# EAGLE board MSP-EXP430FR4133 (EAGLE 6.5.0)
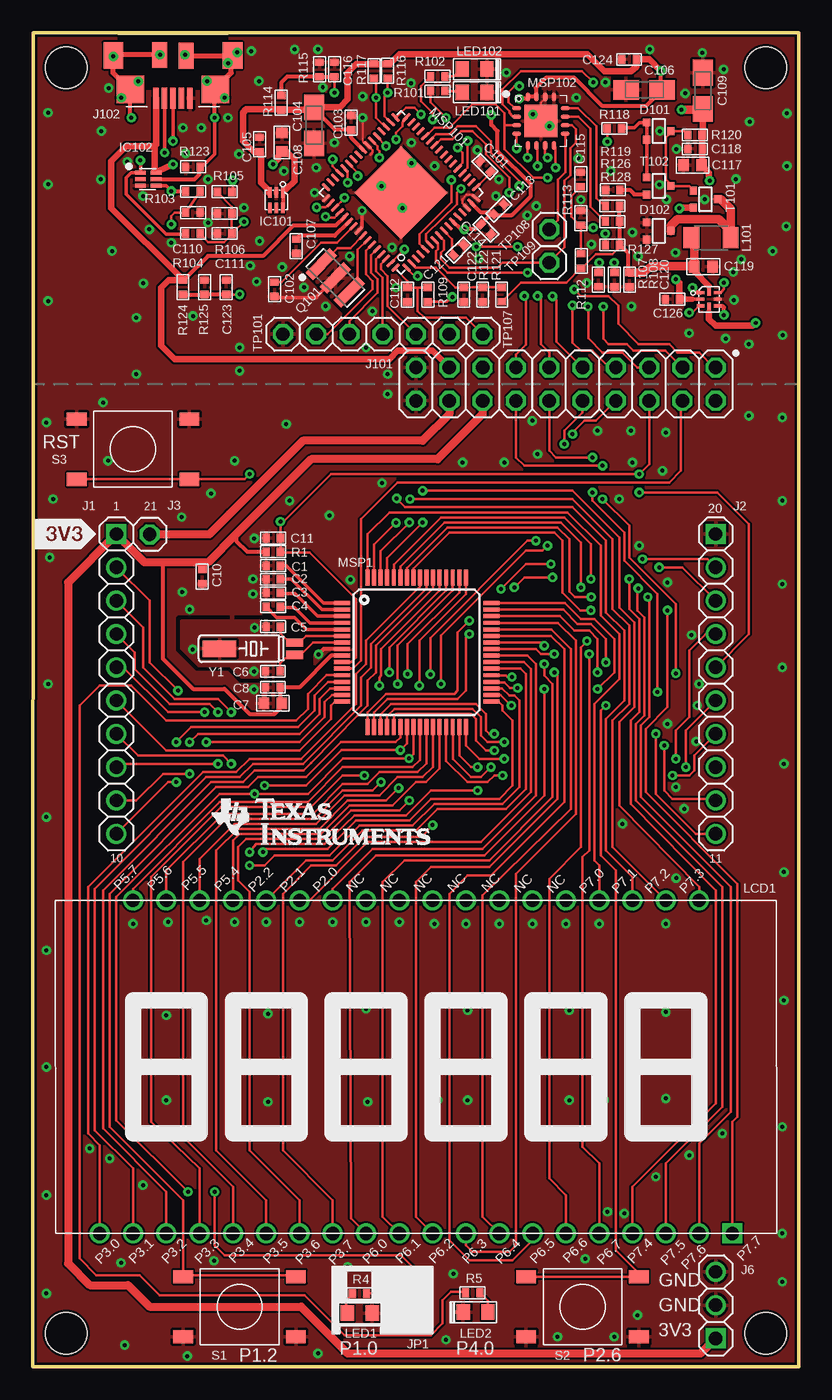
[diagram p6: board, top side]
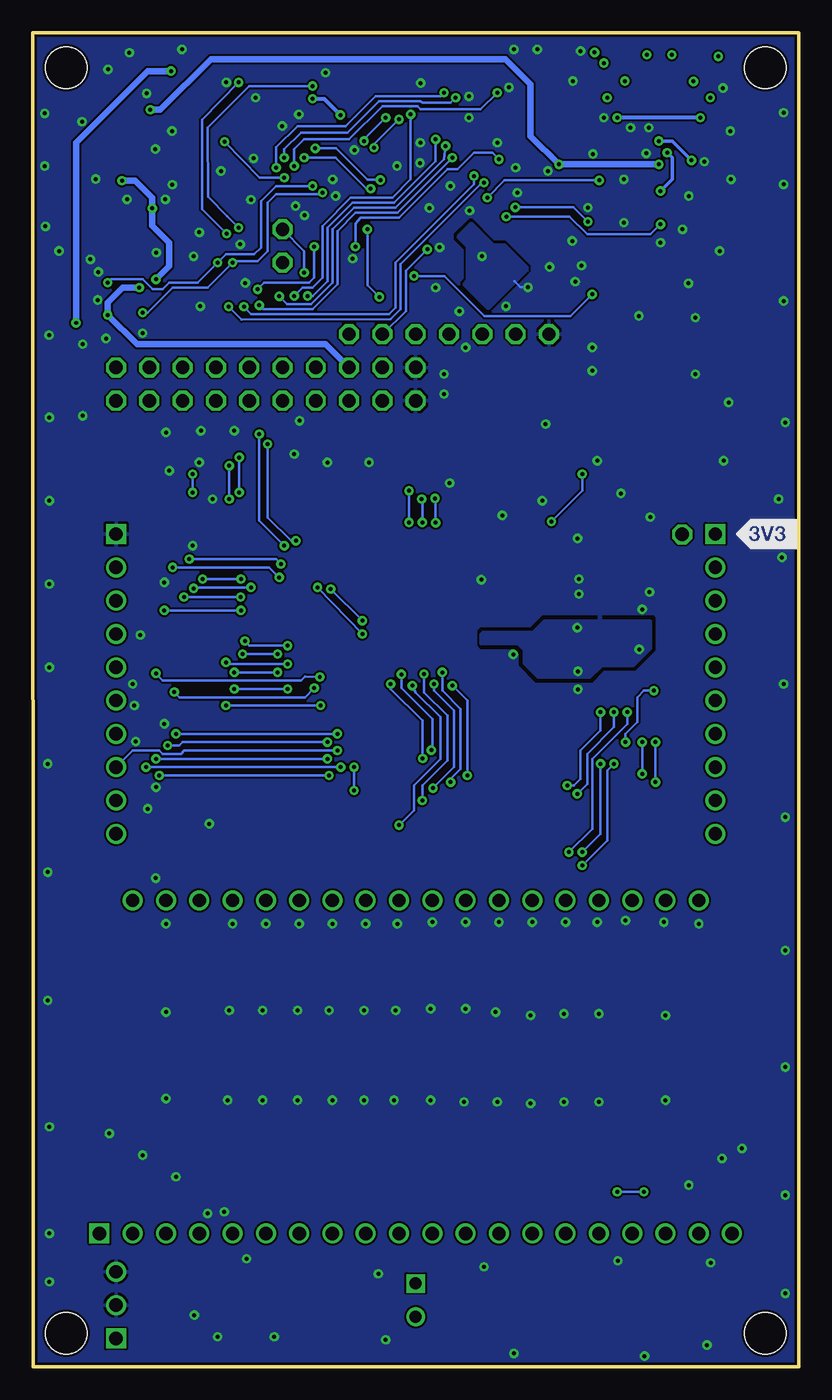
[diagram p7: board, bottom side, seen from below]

Size 58.45 x 101.73 mm. Coordinates in mm from the lower left corner, seen from the top.
Outline: 0,0 58.42,0 58.45,101.73 0.03,101.73 0,0
Copper layers (1*16): Top 0.0178mm / dielectric 12mil / Bottom 0.0178mm
Design rules "default": minimum track width 6mil, minimum drill 12mil, track to track 6mil, track to pad 6mil, pad to pad 6mil, via to via 8mil, smd to smd 0mil, copper to edge 8mil, drill to drill 8mil, minimum pad ring 10mil, minimum via ring 8mil, stop-mask expansion 3mil, vias tented up to drill 15mil, thermal gap 8mil
tRestrict: area 20.5,80.4 to 26.3,87.5; area 10.9,52.2 to 24.5,57.3
bRestrict: area 20.5,80.4 to 26.3,87.5; area 10.9,52.2 to 24.5,57.3

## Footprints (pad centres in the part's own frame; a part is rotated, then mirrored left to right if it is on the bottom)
C0402 = smd 0.55 x 0.65: 1 -0.55,0; 2 0.55,0
C0603 = smd 0.8 x 0.9: 1 -0.7,-0.05; 2 0.7,-0.05
A/3216-18R = smd 1.95 x 1.5: + 1.375,0; - -1.375,0
SOT323 = smd 0.6 x 0.55: 1 -0.65,-0.825; 2 0.65,-0.825; 3 0,1.025
WSON_DSE = smd 0.25 x 0.8: 1 0,0; 2 0.5,0; 3 1,0; 5 0.5,1.15; 6 0,1.15; P4 1,1.15
SON(DRY)6 = smd 0.81 x 0.305: 1 -0.1,0; 2 -0.1,-0.5; 3 -0.1,-1; 4 1.1,-1; 5 1.1,-0.5; 6 1.1,0
UQFN_RSE = smd 0.25 x 0.58: 1 -0.5,-0.65; 2 0,-0.65; 3 0.5,-0.65; 5 0.5,0.65; 6 0,0.65; 7 -0.5,0.65 | smd 0.58 x 0.25: 4 0.55,0; 8 -0.55,0
PINHEAFER1X10 = drill 1.016 square: 1 -11.43,0 | drill 1.016: 2 -8.89,0; 3 -6.35,0; 4 -3.81,0; 5 -1.27,0; 6 1.27,0; 7 3.81,0; 8 6.35,0; 9 8.89,0; 10 11.43,0
1X01 = drill 1.016 octagon: 1 0,0
PINHEADER1X3 = drill 1.016 square: 1 -2.54,0 | drill 1.016: 2 0,0; 3 2.54,0
2X10 = drill 1.016 octagon: 1 -11.43,-1.27; 2 -11.43,1.27; 3 -8.89,-1.27; 4 -8.89,1.27; 5 -6.35,-1.27; 6 -6.35,1.27; 7 -3.81,-1.27; 8 -3.81,1.27; 9 -1.27,-1.27; 10 -1.27,1.27; 11 1.27,-1.27; 12 1.27,1.27; 13 3.81,-1.27; 14 3.81,1.27; 15 6.35,-1.27; 16 6.35,1.27; 17 8.89,-1.27; 18 8.89,1.27; 19 11.43,-1.27; 20 11.43,1.27
EZFET_UX62M-B-5P = smd 0.42 x 1.6: 1 1.3,1.3; 2 0.65,1.3; 3 0,1.3; 4 -0.65,1.3; 5 -1.3,1.3 | smd 2.1 x 2.1: S1 -3.25,0.65; S2 3.25,0.65 | smd 1.5 x 2: S3 -4.55,-1.95; S4 4.55,-1.95 | smd 1.144 x 1.949: S5 -1.016,-1.93; S6 1.016,-1.981
JUMPER-2.54 = drill 0.914 square: 1 0,-1.27 | drill 0.914: 2 0,1.27
L3216C = smd 1.2 x 1.6: 1 -1.5,0; 2 1.5,0
FH1138P = drill 1.016 square: 1 25.4,0 | drill 1.016: 2 22.86,0; 3 20.32,0; 4 17.78,0; 5 15.24,0; 6 12.7,0; 7 10.16,0; 8 7.62,0; 9 5.08,0; 10 2.54,0; 11 0,0; 12 -2.54,0; 13 -5.08,0; 14 -7.62,0; 15 -10.16,0; 16 -12.7,0; 17 -15.24,0; 18 -17.78,0; 19 -20.32,0; 20 -22.86,0; 21 -20.32,25.4; 22 -17.78,25.4; 23 -15.24,25.4; 24 -12.7,25.4; 25 -10.16,25.4; 26 -7.62,25.4; 27 -5.08,25.4; 28 -2.54,25.4; 29 0,25.4; 30 2.54,25.4; 31 5.08,25.4; 32 7.62,25.4; 33 10.16,25.4; 34 12.7,25.4; 35 15.24,25.4; 36 17.78,25.4; 37 20.32,25.4; 38 22.86,25.4
LED0805 = smd 1 x 1.2: A 1.052,0.102; C -0.848,0.102
LQFP64 = smd 1.2 x 0.3: 1 -5.649,3.623; 2 -5.649,3.123; 3 -5.649,2.623; 4 -5.649,2.123; 5 -5.649,1.623; 6 -5.649,1.123; 7 -5.649,0.623; 8 -5.649,0.123; 9 -5.649,-0.377; 10 -5.649,-0.877; 11 -5.649,-1.377; 12 -5.649,-1.877; 13 -5.649,-2.377; 14 -5.649,-2.877; 15 -5.649,-3.377; 16 -5.649,-3.877; 33 5.751,-3.877; 34 5.751,-3.377; 35 5.751,-2.877; 36 5.751,-2.377; 37 5.751,-1.877; 38 5.751,-1.377; 39 5.751,-0.877; 40 5.751,-0.377; 41 5.751,0.123; 42 5.751,0.623; 43 5.751,1.123; 44 5.751,1.623; 45 5.751,2.123; 46 5.751,2.623; 47 5.751,3.123; 48 5.751,3.623 | smd 0.3 x 1.2: 17 -3.699,-5.827; 18 -3.199,-5.827; 19 -2.699,-5.827; 20 -2.199,-5.827; 21 -1.699,-5.827; 22 -1.199,-5.827; 23 -0.699,-5.827; 24 -0.199,-5.827; 25 0.301,-5.827; 26 0.801,-5.827; 27 1.301,-5.827; 28 1.801,-5.827; 29 2.301,-5.827; 30 2.801,-5.827; 31 3.301,-5.827; 32 3.801,-5.827; 49 3.801,5.573; 50 3.301,5.573; 51 2.801,5.573; 52 2.301,5.573; 53 1.801,5.573; 54 1.301,5.573; 55 0.801,5.573; 56 0.301,5.573; 57 -0.199,5.573; 58 -0.699,5.573; 59 -1.199,5.573; 60 -1.699,5.573; 61 -2.199,5.573; 62 -2.699,5.573; 63 -3.199,5.573; 64 -3.699,5.573
RGC64 = smd 0.825 x 0.28: 1 -4.36,3.75; 2 -4.36,3.25; 3 -4.36,2.75; 4 -4.36,2.25; 5 -4.36,1.75; 6 -4.36,1.25; 7 -4.36,0.75; 8 -4.36,0.25; 9 -4.36,-0.25; 10 -4.36,-0.75; 11 -4.36,-1.25; 12 -4.36,-1.75; 13 -4.36,-2.25; 14 -4.36,-2.75; 15 -4.36,-3.25; 16 -4.36,-3.75; 33 4.36,-3.75; 34 4.36,-3.25; 35 4.36,-2.75; 36 4.36,-2.25; 37 4.36,-1.75; 38 4.36,-1.25; 39 4.36,-0.75; 40 4.36,-0.25; 41 4.36,0.25; 42 4.36,0.75; 43 4.36,1.25; 44 4.36,1.75; 45 4.36,2.25; 46 4.36,2.75; 47 4.36,3.25; 48 4.36,3.75 | smd 0.28 x 0.825: 17 -3.75,-4.36; 18 -3.25,-4.36; 19 -2.75,-4.36; 20 -2.25,-4.36; 21 -1.75,-4.36; 22 -1.25,-4.36; 23 -0.75,-4.36; 24 -0.25,-4.36; 25 0.25,-4.36; 26 0.75,-4.36; 27 1.25,-4.36; 28 1.75,-4.36; 29 2.25,-4.36; 30 2.75,-4.36; 31 3.25,-4.36; 32 3.75,-4.36; 49 3.75,4.36; 50 3.25,4.36; 51 2.75,4.36; 52 2.25,4.36; 53 1.75,4.36; 54 1.25,4.36; 55 0.75,4.36; 56 0.25,4.36; 57 -0.25,4.36; 58 -0.75,4.36; 59 -1.25,4.36; 60 -1.75,4.36; 61 -2.25,4.36; 62 -2.75,4.36; 63 -3.25,4.36; 64 -3.75,4.36 | smd 5 x 5: TP 0,0
RSA16 = smd 0.7 x 0.35: 1 -1.85,0.975; 2 -1.85,0.325; 3 -1.85,-0.325; 4 -1.85,-0.975; 9 1.85,-0.975; 10 1.85,-0.325; 11 1.85,0.325; 12 1.85,0.975 | smd 0.35 x 0.7: 5 -0.975,-1.85; 6 -0.325,-1.85; 7 0.325,-1.85; 8 0.975,-1.85; 13 0.975,1.85; 14 0.325,1.85; 15 -0.325,1.85; 16 -0.975,1.85 | smd 2.5 x 2.5: TP 0,0
CSTCR4M = smd 0.8 x 2.6: 1 -1.5,0; 2 0,0; 3 1.5,0
R0402 = smd 0.55 x 0.65: 1 -0.55,0; 2 0.55,0
T062S = smd 1.5 x 1: 1 -4.3,2.3; 2 4.3,2.3; 3 -4.3,-2.3; 4 4.3,-2.3
MOUNTHOLE_125MIL = hole 3.175: 0,0
MS3V-T1R = smd 0.635 x 1.27: P1 -0.47,-4.43; P2 0.47,-4.43 | smd 1.27 x 2.54: P3 0,1.3

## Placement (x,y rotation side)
C1  100n  [C0402]  18.34,61.09 180 top
C2  100n  [C0402]  18.34,60.05 180 top
C3  100n  [C0402]  18.34,59 180 top
C4  1u  [C0402]  18.34,57.96 180 top
C5  12p  [C0402]  18.34,56.44 180 top
C6  12p  [C0402]  18.31,53.04 180 top
C7  10u  [C0603]  18.31,50.55 180 top
C8  100n  [C0402]  18.31,51.82 180 top
C10  100n  [C0402]  12.93,60.25 270 top
C11  1n  [C0402]  18.34,63.2 180 top
C101  470n  [C0402]  34.51,91.53 135 top
C102  220n  [C0402]  18.44,82.17 270 top
C103  100n  [C0402]  24.28,94.87 90 top
C104  10u  [A/3216-18R]  21.46,94.67 90 top
C105  100n  [C0402]  17.3,93.22 90 top
C106  4.7u  [A/3216-18R]  46.63,97.38 0 top
C107  220n  [C0402]  20.09,85.45 270 top
C108  1u  [C0603]  18.95,93.37 90 top
C109  4.7u  [A/3216-18R]  51.11,97.31 270 top
C110  10p  [C0402]  12.22,88.01 0 top
C111  10p  [C0402]  14.63,86.42 180 top
C112  1n  [C0402]  28.58,81.76 270 top
C113  100n  [C0402]  35.55,88.27 45 top
C114  100n  [C0402]  34.57,86.74 315 top
C115  32p  [C0402]  41.81,90.55 270 top
C116  32p  [C0402]  23.01,98.93 270 top
C117  4.7u  [C0603]  50.33,91.57 180 top
C118  100n  [C0402]  50.51,92.88 180 top
C119  4.7u  [C0603]  51.16,83.93 0 top
C120  100n  [C0402]  45.52,82.9 270 top
C121  100n  [C0402]  32.48,85.16 45 top
C122  32p  [C0402]  32.88,81.76 90 top
C123  32p  [C0402]  14.76,82.32 270 top
C124  100n  [C0402]  45.49,99.7 180 top
C126  100n  [C0402]  48.79,81.41 180 top
D101  BAS40-05  [SOT323]  47.65,94.23 270 top
D102  BAS40-05  [SOT323]  47.65,86.61 270 top
DRAW1  [LOGO-ROCKET-10X7MM-BRD]  3.86,81.8 65 top
DRAW3  [LOGO-ROCKET-10X7MM-BRD]  34.15,38.62 7 top
IC101  [WSON_DSE]  19.08,89.53 180 top
IC102  TPD4E004DRYR  [SON(DRY)6]  8.31,91.06 0 top
IC103  TS5A21366RSER  [UQFN_RSE]  51.59,81.41 270 top
J1  [PINHEAFER1X10]  6.38,52.07 270 top
J2  [PINHEAFER1X10]  52.1,52.07 270 top
J3  TEST_PIN2  [1X01]  8.92,63.47 0 top
J6  [PINHEADER1X3]  52.1,4.7 90 top
J101  [2X10]  40.67,74.93 180 top
J102  Micro-USB  [EZFET_UX62M-B-5P]  10.69,98.04 180 top
JP1  [JUMPER-2.54]  29.24,5.08 180 top
L101  2u2  [L3216C]  51.73,86.1 180 top
LCD1  [FH1138P]  27.97,10.16 0 top
LED1  Red  [LED0805]  25.04,4.19 180 top
LED2  Green  [LED0805]  33.68,4.06 0 top
LED101  Red  [LED0805]  33.81,97.28 180 top
LED102  Green  [LED0805]  33.81,99.06 180 top
MSP1  MSP430FR4x  [LQFP64]  29.24,54.61 0 top
MSP101  MSP430F5528IRGC  [RGC64]  28.09,89.54 135 top
MSP102  MSP430G2452IRSA16R  [RSA16]  38.76,95 0 top
Q101  PIEZO_CSTCR4M00G15L99  [CSTCR4M]  23.08,83.02 315 top
R1  47k  [R0402]  18.34,62.15 0 top
R4  470  [R0402]  24.92,5.59 180 top
R5  470  [R0402]  33.55,5.64 0 top
R101  470  [R0402]  30.89,97.28 180 top
R102  470  [R0402]  30.89,98.41 180 top
R103  27  [R0402]  12.22,89.63 0 top
R104  27  [R0402]  12.22,86.42 0 top
R105  1k4  [R0402]  14.63,89.6 0 top
R106  1M  [R0402]  14.63,87.95 180 top
R107  47k  [R0402]  43.15,82.91 270 top
R108  47k  [R0402]  44.37,82.91 270 top
R109  47k  [R0402]  30.14,81.76 270 top
R112  220k  [R0402]  41.84,84.33 90 top
R113  220k  [R0402]  41.81,87.6 90 top
R114  220k  [R0402]  18.95,96.39 90 top
R115  220k  [R0402]  21.87,98.93 90 top
R116  4k7  [R0402]  27.06,98.82 270 top
R117  4k7  [R0402]  26.03,98.82 270 top
R118  820  [R0402]  44.37,94.42 180 top
R119  0  [R0402]  44.24,89.75 180 top
R120  470  [R0402]  50.51,93.94 180 top
R121  220k  [R0402]  35.78,81.76 90 top
R122  220k  [R0402]  34.32,81.76 270 top
R123  33k  [R0402]  12.22,91.5 180 top
R124  240k  [R0402]  11.46,82.32 270 top
R125  150k  [R0402]  13.11,82.32 90 top
R126  2k2  [R0402]  44.22,88.52 180 top
R127  3k3  [R0402]  44.22,85.55 180 top
R128  6k8  [R0402]  44.22,87.33 180 top
S1  T062S  [T062S]  15.77,4.57 180 top
S2  T062S  [T062S]  41.94,4.57 180 top
S3  T062S  [T062S]  7.65,69.98 0 top
T101  DMG1013UW  [SOT323]  51.21,89.03 270 top
T102  BC850CW-115  [SOT323]  47.65,90.04 270 top
TP101  TEST_PIN2  [1X01]  19.08,78.74 0 top
TP102  TEST_PIN2  [1X01]  21.62,78.74 0 top
TP103  TEST_PIN2  [1X01]  24.16,78.74 0 top
TP104  TEST_PIN2  [1X01]  26.7,78.74 0 top
TP105  TEST_PIN2  [1X01]  29.24,78.74 0 top
TP106  TEST_PIN2  [1X01]  31.78,78.74 0 top
TP107  TEST_PIN2  [1X01]  34.32,78.74 0 top
TP108  TEST_PIN2  [1X01]  39.4,86.74 0 top
TP109  TEST_PIN2  [1X01]  39.4,84.2 0 top
U$2  MOUNTHOLE_125MIL  [MOUNTHOLE_125MIL]  2.57,2.54 0 top
U$3  MOUNTHOLE_125MIL  [MOUNTHOLE_125MIL]  2.57,99.06 0 top
U$4  [LOGO16_TPLACE]  13.55,39.64 0 top
U$5  MOUNTHOLE_125MIL  [MOUNTHOLE_125MIL]  55.91,2.54 0 top
U$6  MOUNTHOLE_125MIL  [MOUNTHOLE_125MIL]  55.91,99.06 0 top
U$7  SILK_3V3_TAG  [SILK_3V3_TAG]  0.03,62.36 0 top
U$8  SILK_FR4133_REAR_REV02  [SILK_FR4133_REAR_REV02]  0.03,0.13 0 top
Y1  32.768kHz  [MS3V-T1R]  15.54,54.76 90 top

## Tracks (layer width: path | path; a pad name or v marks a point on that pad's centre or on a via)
5V
  Top 0.152: 8.92,63.5 J3.1
  Top 0.61: J101.18 31.78,72.64 29.74,70.61 20.6,70.61 15.01,65.02 13.46,63.48 J3.1
+3V3
  Top 0.203: 19.01,50.36 C7.1
  Top 0.305: MSP1.9 22.76,54.23 20.35,51.82 C8.1 18.86,50.47 C7.1 19.01,50.57 | 15.52,63.5 15.52,62.98 16.35,62.15 R1.1 | 10.06,61.34 9.93,61.21 9.93,53.98 12.22,51.69 14.63,51.69 16.54,49.78 18.44,49.78 19.01,50.36 | C10.1 12.93,61.34
  Top 0.61: J6.1 50.95,1.02 24.03,1.02 20.47,4.57 8.92,4.57 7.26,6.22 4.34,6.22 2.69,7.87 2.69,59.82 J1.1 8.53,61.34 10.06,61.34 12.93,61.34 13.36,61.34 15.52,63.5 21.23,69.22 30.89,69.22 34.32,72.64 J101.16
EZFET_AVBUS  (via drill 0.3)
  Top 0.203: v29.36,83.19 29.11,83.19 28.52,83.77 MSP101.1 | C123.2 15.38,81.77 v15.77,81.79
  Top 0.305: R124.2 12.96,81.77 12.98,81.79 13.12,81.79 | C123.2 R125.1 13.12,81.79 | 13.23,81.79 13.12,81.79
  Bottom 0.203: v29.36,83.19 27.03,83.19 23.98,80.14 17.42,80.14 v15.77,81.79
EZFET_AVCC  (via drill 0.3)
  Top 0.152: 38.51,93.08 38.51,93.09 MSP102.6
  Top 0.203: 23.01,98.28 v23.01,97.16 | v38.51,91.57 38.51,93.08
  Top 0.305: 23.01,98.28 C116.2 | C116.2 23.01,98.43 22.97,98.38 R115.1 19.41,98.38 18.95,97.92 R114.2 | 23.01,98.3 C116.2 | C116.2 | R114.2
  Bottom 0.203: v23.01,97.16 24.28,95.89 28.85,95.89 29.11,96.14 31.78,96.14 34.32,93.6 37.74,93.6 38.51,92.84 v38.51,91.57
EZFET_AVCCOUT  (via drill 0.3)
  Top 0.152: 36.73,96.01 36.86,96.01 MSP102.1
  Top 0.203: R113.1 41.81,85.98 41.81,84.96 41.83,84.96 R112.2 | R113.1 42.03,86.87 v42.75,86.87 | 36.73,96.01 36.27,96.44 36.27,97.21 36.73,97.66 v37.11,97.66 | 41.78,89.97 41.78,89.94 41.83,89.89 41.86,89.92 | 41.86,89.82 41.86,89.92 | 41.86,89.92 41.86,89.95 41.83,89.97 | C115.2 41.79,90 41.07,89.28 41.07,87.71 41.68,87.1 41.77,86.84 R113.1
  Top 0.508: C115.2 41.78,89.97
  Bottom 0.203: v37.11,97.66 41.94,97.66 45.11,94.49 45.09,89.23 43.61,87.76 v42.75,86.87
EZFET_AVCCOUT2ADC
  Top 0.203: R121.2 34.21,82.31 R122.1 33.59,82.31 C122.2 32.55,82.31 32.25,82.31 30.76,83.82 29.21,83.82 MSP101.2
EZFET_DCDCCAL0
  Top 0.203: R126.2 43.7,88.39 43.33,88.77 42.98,89.13 42.98,94.62 41.6,95.97 MSP102.12
EZFET_DCDCCAL1  (via drill 0.3)
  Top 0.203: MSP102.2 36.85,95.38 36.6,95.38 36.35,95.63 36.35,95.76 35.84,96.27 35.84,97.41 37.24,98.81 41.88,98.81 v42.75,97.94 | R127.2 43.67,85.51 43.66,85.88 43.66,86.34 43.69,86.36 43.66,86.36 v43.66,86.41
  Bottom 0.203: v42.75,97.94 45.54,95.1 45.54,88.27 v43.66,86.41
EZFET_DCDCCAL2
  Top 0.203: R128.2 42.55,88.45 42.55,94.41 41.63,95.33 40.63,95.33 MSP102.11
EZFET_DCDCIO0  (via drill 0.3)
  Top 0.203: v36.91,92.91 36.91,93.15 MSP102.4 | v31.93,90.5 31.93,88.8 29.49,86.36 29.49,85.66 MSP101.5
  Bottom 0.203: v36.91,92.91 35.31,92.91 32.92,90.53 32.16,90.53 v31.93,90.5
EZFET_DCDCIO1  (via drill 0.3)
  Top 0.203: 30.12,85.74 MSP101.6 30,85.86 30,86.36 32.35,88.66 32.36,88.67 32.36,89.53 v32.66,89.84 | v37.74,92.2 37.74,93.11 MSP102.5
  Bottom 0.203: v37.74,92.2 35.33,92.2 32.97,89.84 v32.66,89.84
EZFET_DCDCPULSE  (via drill 0.3)
  Top 0.203: R118.2 43.82,93.72 v43.82,93.42 | v39.27,90.68 38.18,90.68 35.97,92.84 35.97,94.74 | 35.97,94.74 35.97,95.61 35.31,96.27 33.55,96.27 31.78,94.49 30.63,94.49 30,93.86 MSP101.28 | 35.97,94.74 36.04,94.67 MSP102.3
  Bottom 0.203: v39.27,90.68 41.15,90.68 v43.82,93.42
EZFET_DCDCRST  (via drill 0.3)
  Top 0.203: MSP101.7 30.66,85.9 30.91,85.65 30.91,85.24 30.76,85.09 30.76,84.33 31.65,83.44 v37.74,83.44 | 40.78,93.98 MSP102.9 40.61,91.08 40.06,90.53 40.06,87.43 TP108.1 | TP108.1 39.42,86.77 39.37,86.82 TP108.1
  Top 0.305: TP108.1
  Bottom 0.203: TP108.1 | TP108.1 37.74,85.09 v37.74,83.44
EZFET_DCDCTEST
  Top 0.203: MSP101.8 31,86.25 31.37,85.88 31.37,85.19 31.14,84.96 31.14,84.46 31.78,83.82 35.46,83.82 35.84,84.2 TP109.1 39.8,84.61 40.56,85.37 40.56,90.45 41,90.88 41,92.91 41.43,93.34 41.43,94.36 41.12,94.67 40.74,94.67 40.67,94.74 40.67,94.62 MSP102.10
EZFET_DM  (via drill 0.3)
  Top 0.203: J102.2 10.04,96.66
  Top 0.254: IC102.4 10.17,90.06 v10.57,89.66 | 10.04,96.66 v10.06,92.58
  Top 0.305: v10.57,89.66 11.58,89.66 11.61,89.63 R103.1
  Bottom 0.254: v10.57,89.66 9.68,90.55 9.68,92.2 v10.06,92.58
EZFET_DP  (via drill 0.3)
  Top 0.254: v8.2,92 v8.21,92.01 IC102.1 7.52,91.06 7.14,90.68 7.14,89.41 10.19,86.36 11.5,86.36 R104.1 | J102.3 v10.69,93.47
  Bottom 0.254: v10.69,93.47 9.68,93.47 v8.2,92
EZFET_HOSTSCL  (via drill 0.3)
  Top 0.152: MSP101.35 26.95,94.62 26.95,94.61
  Top 0.203: 26.95,94.61 26.83,94.61 26.19,95.25 v26.19,96.77 26.19,98.25 | v39.27,92.2 39.09,92.36 MSP102.7
  Top 0.305: 26.19,98.25 R117.2
  Bottom 0.203: v26.19,96.77 26.57,96.39 28.73,96.39 28.85,96.52 32.03,96.52 34.44,94.11 38,94.11 39.27,92.84 v39.27,92.2
EZFET_HOSTSDA  (via drill 0.3)
  Top 0.203: MSP101.34 27.28,94.92 26.82,95.38 26.82,96.9 v27.08,97.16 27.08,98.16 R116.2 | MSP102.8 39.88,92.98 v39.88,91.44
  Bottom 0.203: v27.08,97.16 27.33,96.9 32.28,96.9 34.57,94.62 38.25,94.62 39.88,92.99 v39.88,91.44
EZFET_LED0  (via drill 0.3)
  Top 0.203: MSP101.20 33.17,91.44 v33.17,93.47 | v31.52,95.25 30.34,96.44 R101.2
  Bottom 0.203: v33.17,93.47 33.17,93.6 v31.52,95.25
EZFET_LED1  (via drill 0.3)
  Top 0.203: R102.2 30.24,98.28 29.62,97.66 29.62,96.52 30.51,95.63 v30.51,95.12 | MSP101.21 32.41,91.44 32.79,91.82 32.79,92.58 v32.41,92.96
  Bottom 0.203: v32.41,92.96 32.41,93.22 v30.51,95.12
EZFET_NC_TMSC  (via drill 0.3)
  Top 0.203: J101.1 51.97,76.2 50.83,77.34 49.17,77.34 48.54,77.98 46.2,77.98 44.65,79.53 44.65,80.92 43.92,81.66 41.81,81.66 v41.3,82.17 | MSP101.45 22.89,91.57 v22.89,92.08 | 36.98,85.47 v36.98,85.42 36.98,85.34 36.93,85.42 v33.83,85.42
  Bottom 0.203: v22.89,92.08 23.39,92.58 24.79,92.58 26.06,91.31 26.82,91.31 30.51,87.63 33.43,87.63 33.83,87.17 v33.83,85.42 | v36.98,85.42 36.98,83.06 37.36,82.68 40.79,82.68 v41.3,82.17
EZFET_PU.0/DP  (via drill 0.3)
  Top 0.152: 22.76,88.77 MSP101.50
  Top 0.203: v16.1,87.33 15.33,86.55 C111.1 | R105.1 15.18,88.48 R106.1 15.18,87.47 C111.1 | R104.2 13.39,85.78 14.58,85.78 15.15,86.35 C111.1 | 22.76,88.77 22.5,88.52 22.45,88.52 22.35,88.42 v21.64,88.42
  Bottom 0.203: v16.1,87.33 17.2,88.42 v21.64,88.42
EZFET_PU.1/DM  (via drill 0.3)
  Top 0.203: R103.2 12.74,89.56 C110.1 10.82,88.01 10.57,87.76 v10.57,87.12 | MSP101.52 23.01,87.63 22.5,87.63 v22.33,87.71
  Bottom 0.203: v22.33,87.71 17.5,87.71 16.15,86.36 11.33,86.36 v10.57,87.12
EZFET_PUR  (via drill 0.3)
  Top 0.203: MSP101.51 23.52,88.85 v23.77,89.15 | v15.24,90.48 15.25,89.7 R105.2
  Bottom 0.203: v15.24,90.48 22.45,90.48 v23.77,89.15
EZFET_RST
  Top 0.203: MSP101.64 27.79,83.62 28.6,82.8 28.6,82.37 C112.1 R109.1 | TP107.1 33.05,80.01 29.87,80.01 29.36,80.52 29.36,82.3 30.12,82.3 R109.1 | R109.1 | R109.1 30.12,82.3
EZFET_SBWTCK  (via drill 0.3)
  Top 0.203: MSP101.44 23.75,91.39 24.03,91.11 v24.03,90.3 | J101.3 48.26,77.47 45.82,77.47 45.31,77.98 43.92,77.98 43.51,78.38 v43.51,80.85
  Bottom 0.203: v24.03,90.3 24.28,90.17 30.38,84.07 30.38,80.65 31.14,79.88 42.52,79.86 v43.51,80.85
EZFET_SBWTDIO  (via drill 0.3)
  Top 0.203: MSP101.43 24.79,91.06 v24.79,90.81 | J101.5 46.13,76.2 44.98,77.34 43.46,77.34 42.37,78.44 42.37,80.82 v42.34,80.85
  Bottom 0.203: v24.79,90.81 24.79,90.17 30.76,84.2 30.76,80.77 31.27,80.26 41.78,80.29 v42.34,80.85
EZFET_SHIELD  (via drill 0.3)
  Top 0.152: 14,97.03 13.87,96.9 13.87,96.77
  Top 0.203: 7.44,95.12 7.52,95.12 v7.52,95.25 | 7.44,96.77 7.39,96.77 | 7.39,96.77 7.39,97.28 | v6.76,96.77 7.39,96.77 | v14.63,96.77 13.87,96.77
  Top 0.254: R123.1 12.92,91.5 13.87,92.46 v13.87,95.25
  Top 0.305: IC102.5 12.21,90.56 12.34,90.55 12.73,90.93 12.73,91.34 R123.1 12.73,91.23 | 7.44,95.12 7.44,96.77 | v13.87,95.25 13.87,96.77
  Top 0.381: J102.S2 7.41,97.39 6.12,98.68 6.12,99.95 6.14,99.97 J102.S4 | J102.S4 v6.14,99.93 v6.15,99.92 | 14,97.03 14,97.45 | J102.S2 7.44,97.33 7.39,97.28 | v8.05,98.02 8.05,98 J102.S2 | v13.28,98.04 v13.29,98.04 J102.S1 14,97.45 | 14,97.45 14,97.54 15.14,98.68 15.14,99.16 v14.88,99.42 14.88,99.64 J102.S3 | v15.6,100.23 15.6,99.97 J102.S3 | J102.S3 15.22,99.97 J102.S5 11.68,99.97 v11.61,100.05 | 9.68,100.05 6.2,100.05 J102.S4
  Top 0.406: J102.S6 9.68,100.05 v9.7,100.05
  Bottom 0.305: v7.52,95.25 v13.87,95.25
EZFET_TCK  (via drill 0.3)
  Top 0.203: v28.35,85.22 27.31,84.18 MSP101.63
  Bottom 0.203: v28.35,85.22 29.97,83.59 29.97,80.49 TP106.1 | TP106.1
EZFET_TDI
  Top 0.203: MSP101.61 26.59,84.86 26.19,84.46 26.19,83.57 26.7,83.06 TP104.1 | TP104.1
EZFET_TDO
  Top 0.203: TP103.1 24.16,79.76 26.31,81.92 26.31,82.93 25.81,83.44 25.81,84.77 MSP101.60
EZFET_TEST
  Top 0.203: 25.93,85.6 25.92,85.6 MSP101.59 25.43,85.1 25.43,83.31 25.93,82.8 25.93,82.17 22.5,78.74 TP102.1
EZFET_TMS
  Top 0.203: MSP101.62 26.95,84.46 26.57,84.07 26.57,83.69 27.08,83.19 27.08,80.9 TP105.1
EZFET_UARTCTS  (via drill 0.3)
  Top 0.203: 28.35,95.12 28.22,94.87 28.22,94.62 27.71,94.11 v27.71,93.6 | 37.62,81.53 v37.49,81.66 37.62,81.53 | J101.13 36.86,77.19 37.62,77.95 37.62,81.53
  Top 0.254: MSP101.32 28.49,95.27 28.35,95.12
  Bottom 0.203: v27.71,93.6 27.71,91.95 30.89,88.77 34.06,88.77 35.97,86.87 35.97,82.8 37.11,81.66 v37.49,81.66
EZFET_UARTRTS  (via drill 0.3)
  Top 0.203: 27.69,95.27 27.71,95.25 | 27.84,95.12 27.71,95.25 | 27.71,95.25 28.47,96.01 29.11,96.01 v29.62,95.5 | J101.11 39.4,77.34 38.76,77.98 38.76,81.41 v38.51,81.66
  Top 0.254: MSP101.33 27.69,95.27
  Bottom 0.203: v29.62,95.5 29.62,90.55 31.01,89.15 34.19,89.15 36.35,87 36.35,83.06 37.11,82.3 37.87,82.3 v38.51,81.66
EZFET_UARTRXD  (via drill 0.3)
  Top 0.203: MSP101.38 26.31,93.09 26.31,92.84 26.44,92.71 v26.44,92.2 | J101.7 43.97,76.2 42.7,77.47 41.81,77.47 41.17,78.11 v41.17,80.95
  Bottom 0.203: v26.44,92.2 30.63,88.01 33.81,88.01 35.2,86.61 35.2,82.55 37.11,80.65 40.87,80.65 v41.17,80.95
EZFET_UARTTXD  (via drill 0.3)
  Top 0.203: MSP101.37 26.25,93.79 v26.95,93.09 | J101.9 39.95,78.18 39.95,81.33 v39.65,81.64
  Bottom 0.203: v26.95,93.09 27.08,92.08 30.76,88.39 33.93,88.39 35.59,86.74 35.59,82.68 37.24,81.03 39.04,81.03 v39.65,81.64
EZFET_V18
  Top 0.203: MSP101.55 24.45,86.96 23.22,85.73 22,85.73 18.99,82.72 C102.1
EZFET_VBUS  (via drill 0.3)
  Top 0.203: 9.3,91.19 9.3,91.06 IC102.6 | 9.55,91.19 IC102.6 | IC102.6 | 51.1,95.66 51.1,95.93 C109.+
  Top 0.254: IC103.2 50.32,81.41
  Top 0.305: MSP101.53 23.11,87.02 19.86,87.02 17.55,84.71 13.36,84.71 11.71,83.06 11.33,83.06 | 19.33,89.79 IC101.1 IC101.6
  Top 0.406: 50.32,81.41 C126.1 49.3,81.41
  Top 0.508: 9.3,93.09 9.3,91.19 | 9.55,91.19 v10.69,91.69 | J101.17 30.51,77.47 27.84,77.47 27.2,76.84 10.82,76.84 9.8,77.85 9.8,82.3 10.38,82.87 R124.1 11.33,83.06 5.99,88.37 5.99,91.95 7.14,93.09 9.3,93.09 | v18.31,91.69 18.69,92.08 18.69,92.33 19.08,92.71 19.04,92.71 C108.1 19.37,92.67 19.96,92.08 19.96,90.42 19.33,89.79 | J102.1 9.39,93.19 9.3,93.09 | 51.1,95.66 51.1,94.01 51.06,93.96 R120.1 C118.1 51.06,91.65 C117.1 51.59,91.06 51.59,90.42 51.61,90.42 v51.64,90.45 | T101.2 49.32,88.38 | 49.32,88.38 49.3,88.39 | v49.33,88.34 49.33,88.37 49.32,88.38 | v49.05,82.93 49.3,82.68 49.3,81.45 C126.1
  Top 0.635: C109.+ 50.62,95.88 50.39,95.86 v49.48,95.86
  Bottom 0.305: 48.87,95.81 48.74,95.86
  Bottom 0.508: v10.69,91.69 v18.31,91.69 20.47,93.85 20.47,97.79 22.38,99.7 44.86,99.7 48.74,95.86 v49.48,95.86 | v51.64,90.45 50.62,90.45 49.33,89.15 v49.33,88.34 49.33,87.02 48.03,85.73 48.03,83.95 v49.05,82.93
EZFET_VCC  (via drill 0.3)
  Top 0.152: MSP101.11 32.03,87.38 32.07,87.34 | 33.86,86.79 C114.1 | 33.43,88.77 MSP101.15
  Top 0.203: 24.66,93.32 MSP101.40 | v32,81.59 31.58,81.21 R109.2 | R116.1 27.08,99.44 | C114.1 34.06,87.12 | 33.86,86.79 34.13,87.06 | 34.95,94.74 34.98,94.77
  Top 0.254: 17.93,89.53 IC101.3 | IC103.4 51.59,80.39
  Top 0.305: MSP101.40 25.19,92.82 24.28,93.73 C103.1 23.05,94.32 21.49,95.89 21.49,96.01 C104.+ | 25.52,99.34 R117.1 25.44,99.31 | 46.17,99.73 C124.1 46.04,99.2 45.99,99.1 | 48.14,97.71 C106.+ | 43.59,98.81 45.69,98.81 45.99,99.1 | 38.42,96.82 38.38,97.03 38.38,97.54 39.14,98.3 41.3,98.3 43.46,96.14 46.76,96.14 47.56,96.93 C106.+ | 38.42,96.82 38.43,96.75 | 33.6,88.61 MSP101.15 | 32.07,87.34 32.66,86.74 v32.92,86.74 33.76,86.74 34.13,87.06 35.08,88.01 | v37.11,96.7 37.64,96.7 MSP102.16 MSP102.15 38.42,96.82 | C106.+ 47.73,97.38 47.9,97.59 v47.9,98.81 | 46.06,99.05 45.99,99.1 | 35.08,88.01 35.38,87.83 36.55,87.83 38,89.28 38,90.17 35.46,92.71 35.46,94.23 34.98,94.72 34.98,94.77 v34.98,95.45 | 35.08,88.01 35.14,88.01 C113.1 | 35.08,88.01 34.19,88.01 33.43,88.77
  Top 0.406: 17.85,89.88 17.93,89.75 17.93,89.53 | 17.42,92.46 17.3,92.46 C105.1 17.3,92.62 16.88,92.62
  Top 0.508: 16.88,92.62 16.03,93.47 16.03,95.63 16.28,95.89 18.91,95.89 R114.1 21.26,95.84 C104.+ 23.42,96.04 24.03,96.65 24.03,98.68 24.66,99.31 25.44,99.31 27,99.31 R116.1 27.26,99.37 27.97,100.08 42.32,100.08 43.59,98.81 45.62,98.81 46.02,99.14 46.02,99.64 | 17.85,89.88 17.42,90.3 17.42,92.46 17.34,92.67 17.35,92.67 | v47.9,98.81 47.02,99.7 C124.1 | v55.14,79.6 55.14,79.63 54.89,79.38 52.1,79.38 51.59,79.88 51.59,80.39
  Bottom 0.203: v32.92,86.74 32.92,82.5 v32,81.59
  Bottom 0.305: v37.11,96.7 36.22,96.7 v34.98,95.45
  Bottom 0.508: v47.9,98.81 49.68,98.81 55.14,93.34 v55.14,79.6
EZFET_VCCEN1  (via drill 0.3)
  Top 0.203: MSP101.26 30.69,93.15 31.14,93.6 32.03,93.6 32.66,94.23 33.55,94.23 34.57,93.22 34.57,92.46 36.35,90.68 v36.35,89.53 | v50.06,80.39 50.32,80.39 50.83,80.91 IC103.3 | R107.1 43.15,83.88 v43.21,84.2
  Bottom 0.203: v36.35,89.53 36.47,89.41 39.9,89.41 40.54,88.77 40.54,85.09 41.3,84.33 43.08,84.33 v43.21,84.2 45.11,82.3 47.78,82.3 49.68,80.39 v50.06,80.39
EZFET_VCCEN2  (via drill 0.3)
  Top 0.203: MSP101.27 30.29,93.51 30.76,93.98 31.78,93.98 32.41,94.62 33.81,94.62 34.95,93.47 34.95,92.58 37.11,90.42 v37.11,90.04 | R108.1 v44.35,84.2 | IC103.7 52.47,81.91 52.73,82.17 v52.73,82.68
  Bottom 0.203: v37.11,90.04 39.9,90.04 41.05,88.9 41.05,85.34 41.55,84.84 43.71,84.84 v44.35,84.2 45.87,82.68 48.03,82.68 48.54,82.17 49.3,82.17 50.06,82.93 52.48,82.93 v52.73,82.68
EZFET_VCCOUT
  Top 0.203: R121.1 35.93,81.37 37.24,82.68 40.69,82.68 41.81,83.81 | 41.81,83.81 41.81,83.82 41.94,83.82 42.95,84.84 44.22,84.84 44.73,85.34 44.73,85.38 R127.1 | 41.81,83.81 R112.1
  Top 0.254: 51.59,82.42 IC103.8
  Top 0.305: R126.1 44.74,88.01 R128.1 R127.1 45.4,84.96 45.4,83.45 C120.1 | 46.63,83.48 46.63,83.45
  Top 0.508: 50.55,83.92 50.55,83.46 51.59,82.42
  Top 0.635: 46.63,83.48 47.19,83.92 50.43,83.92 C119.1 50.46,83.9 50.47,83.9 | L101.2 50.44,85.82 50.44,84.18 50.42,84.18 50.42,84.07 50.55,84.07 50.55,83.92 50.47,83.92 50.47,83.9 | 50.47,83.87 50.47,83.9 | 46.63,83.45 C120.1
EZFET_VCCTARGET  (via drill 0.3)
  Top 0.254: IC103.5 52.21,80.91
  Top 0.305: IC103.1 50.71,81.91 v50.32,82.3 | 52.21,80.91 52.6,80.91 52.73,80.77 v52.73,80.21
  Bottom 0.508: J101.15 36.09,77.98 50.5,77.98 v52.73,80.21 52.73,81.15 51.59,82.3 v50.32,82.3
EZFET_VCORE
  Top 0.203: MSP101.17 34.93,91.07 C101.1
EZFET_VREF
  Top 0.203: C121.1 31.98,84.75 31.98,86 MSP101.9
EZFET_VUSB
  Top 0.305: MSP101.54 23.04,86.25 20.36,86.25 20.09,85.98 | C107.1 20.09,85.98 | 20.09,85.98
EZFET_XT2IN
  Top 0.203: MSP101.57 25.16,86.27 24.23,85.32 23.24,85.32 22.06,84.14 22,84.07
  Top 0.406: Q101.1 22.06,84.08 22.06,84.14
EZFET_XT2OUT
  Top 0.203: MSP101.58 24.79,85.17 24.79,82.8 24.2,82.21
  Top 0.406: Q101.3 24.2,81.96 24.2,82.21
GND  (via drill 0.3)
  Top 0.152: v25.17,95.25 25.17,93.47 25.43,93.22 MSP101.39 | MSP102.TP 38.76,96.39 39.14,96.77 MSP102.14 | 26.79,88.05 26.82,88.01 MSP101.TP 27.2,88.65
  Top 0.203: 33.63,89.31 33.53,89.31 | 33.63,89.31 33.63,89.3 MSP101.16 | MSP101.56 24.83,86.66 | MSP101.39 25.93,92.76 25.93,92.61 25.76,92.43 | MSP101.14 32.79,88.72 32.79,89.05 33.1,89.38 33.53,89.38 33.63,89.31
  Top 0.254: 24.83,86.66 24.86,86.66 25.12,86.92 v25.12,88.16 | Q101.2 22.95,82.9 21.62,81.56
  Top 0.305: 21.62,81.56 18.46,81.53 C102.2 | MSP1.8 22.45,54.73 22.2,54.74 v21.79,54.33
  Bottom 0.203: v20.68,82.32 21.23,82.32 21.72,82.8
  other vias: 10.57,85.73 8.89,86.74 51.08,100.2 41.45,96.77 24.18,84.68 33.91,92.79 35.33,89.28 19.96,100.46 23.01,93.34 53.49,81.36 43.69,97.94 46.18,84.68 45.75,86.51 47.83,94.23 44.09,91.19 52.7,98.93 17.25,98.04 47.07,100.46 35.56,90.55 48.34,89.03 49.1,92.86 8.43,82.63 16.59,83.97 25.17,96.88 28.85,97.89 17.07,82.75 22.35,80.87 19.02,83.87 27.08,74.17 27.41,85.37 30.66,91.57 12.22,80.14 22.12,97.56 5.18,90.55 5.23,94.23 16.66,100.33 5.79,97.51 15.72,92.48 13.36,87.25 11.66,92.53 14.88,95.25 16.1,88.39 8.41,89.28 11.46,94.49 27.71,82.3 47.8,90.14 38.4,88.52 41.61,92.15 42.62,85.6 49.76,97.1 21.62,91.44 41.81,89 7.9,80.01 48.29,71.25 48.41,59.82 45.62,71.37 43.08,71.37 38.1,72.14 1.17,81.28 1.17,90.17 1.17,95.63 21.74,100.46 46.13,3.94 57.18,6.48 57.18,10.16 57.18,53.34 57.18,59.69 57.18,66.04 57.18,72.39 57.2,78.66 57.48,86.97 57.53,91.57 57.53,95.58 54.69,94.95 56.44,85.09 54.64,77.98 54.64,72.52 11.35,64.8 19.33,71.88 46.25,62.61 13.23,34.04 15.39,33.91 17.81,33.91 20.35,33.91 22.89,33.91 25.43,33.91 27.97,33.91 30.63,33.78 33.05,33.78 35.59,33.78 38.13,33.78 40.67,33.78 43.21,33.78 43.84,11.81 45.11,11.68 48.29,33.78 44.98,41.4 22.63,64.92 7.65,33.78 10.31,33.91 10.19,20.32 10.19,26.8 15.27,26.92 15.27,20.19 17.93,20.19 17.93,26.92 20.47,26.8 20.47,20.07 23.14,27.05 23.01,20.19 25.43,27.31 25.55,20.19 28.09,27.31 28.09,20.32 30.76,27.18 30.89,20.32 33.17,27.18 33.17,20.32 35.84,27.18 35.59,20.32 38.25,27.18 38.25,20.32 40.92,27.18 40.92,20.32 43.46,27.18 43.59,20.32 48.29,27.05 48.29,20.45 8.41,13.84 5.87,15.88 4.34,16.64 52.6,17.78 50.06,16.13 47.52,14.48 48.41,49.02 50.6,47.68 49.05,44.2 49.68,42.55 15.39,69.09 19.58,66.04 7.01,1.65 11.79,0.81 21.74,1.02 1.04,5.59 1.04,13.08 1.04,22.86 1.04,31.75 1.04,41.91 1.17,52.07 1.3,61.72 1.04,72.01 40.03,2.29 44.35,2.29 32.08,7.09 24.03,7.62 13.82,8.08 6.73,7.92 42.14,8.23 57.18,18.29 57.3,27.94 57.3,37.72 57.3,45.97 16.79,58.93 16.79,60.07 49.07,37.26 50.83,52.07 50.24,55.8 44.73,66.17 38.51,69.6 35.97,68.96 5.36,73.53 32.79,68.96 1.55,66.17 11.4,59.08 25.43,77.72 27.08,75.69 15.77,77.72 15.77,75.95 7.9,75.69 45.75,68.96 25.91,80.49 48.03,68.33 5.74,69.09 13.59,66.6 50.7,50.42 31.52,2.06 16.89,63.17 11.96,57.76 16.87,51.66 16.87,53.04 12.19,54.71 16.92,56.36 6.05,85.09 19.15,91.19 17.3,85.85 26.59,90.04 28.19,88.37 38.15,95.5 39.42,94.62 21.49,89.53 7.21,91.9 12.85,94.49 13.36,90.55 28.91,91.8 53.64,90.58 37.72,87.81 34.04,84.51 52.86,78.41 49.02,84.96 54.05,84.46 50.06,78.82 53.44,83.49 45.67,80.87 26.64,67.39 24.23,60.02 51.26,89.03 28.88,93.34 36.12,98.68 42.24,82.65
  pour Top: 0.03,101.6 0.03,0 58.45,0 58.45,101.6
  pour Bottom: 0.03,101.6 0.03,0 58.45,0 58.45,101.6
L0
  Top 0.203: LCD1.35 43.21,38.23 42.82,38.61 42.82,50.55 44.73,52.45 44.73,55.88 43.33,57.28 43.33,62.61 40.79,65.15 27.2,65.15 25.54,63.48 MSP1.64
L1  (via drill 0.3)
  Top 0.203: LCD1.36 45.75,37.34 43.71,39.37 43.71,49.4 45.11,50.8 45.11,56.13 43.71,57.53 43.71,62.99 41.15,65.56 28.4,65.56 v27.76,66.22 | MSP1.63 26.04,62.71 27.71,64.39
  Top 0.406: v27.71,64.36 27.71,64.39
  Bottom 0.203: v27.71,64.36 27.71,66.17 v27.76,66.22
L2  (via drill 0.3)
  Top 0.203: v28.78,66.17 41.17,66.17 44.22,63.12 44.22,57.79 45.49,56.52 45.49,50.55 44.22,49.28 44.22,39.62 LCD1.37 | MSP1.62 26.54,62.2 v28.73,64.39
  Bottom 0.203: v28.73,64.39 28.73,66.12 v28.78,66.17
L3  (via drill 0.3)
  Top 0.203: LCD1.38 50.83,36.58 44.73,42.8 44.73,49.15 45.87,50.29 45.87,56.77 44.73,57.91 44.73,63.25 41.17,66.8 v29.74,66.8 | MSP1.61 27.04,61.68 v29.74,64.39
  Bottom 0.203: v29.74,64.39 v29.74,66.8
L4  (via drill 0.3)
  Top 0.203: v42.57,60.07 42.57,62.74 40.54,64.77 31.14,64.77 27.54,61.17 MSP1.60 | LCD1.4 45.75,13.72 52.1,20.07 52.1,36.32 45.62,42.93 45.62,49.28 46.25,49.91 46.25,57.02 45.49,57.79 v45.49,60.07
  Bottom 0.203: v42.57,60.07 v45.49,60.07
L5  (via drill 0.3)
  Top 0.203: v41.81,59.44 41.81,62.87 40.28,64.39 31.39,64.39 28.04,61.03 MSP1.59 | LCD1.3 48.29,15.49 52.6,19.81 52.6,36.58 46,43.18 46,49.02 46.63,49.66 46.63,57.15 46.13,57.66 46.13,59.31 v46.18,59.36
  Bottom 0.203: v41.81,59.44 46.1,59.44 v46.18,59.36
L6  (via drill 0.3)
  Top 0.203: LCD1.2 50.83,17.02 53.24,19.43 53.24,36.58 46.38,43.43 46.38,48.9 47.04,49.56 47.04,58.57 v46.91,58.7 | v42.6,58.7 41.35,58.7 40.92,59.13 40.92,63.12 40.03,64.01 31.65,64.01 28.54,60.9 MSP1.58
  Bottom 0.203: v42.6,58.7 v46.91,58.7
L7  (via drill 0.3)
  Top 0.203: v48.41,57.68 48.41,50.29 46.76,48.64 46.76,43.82 53.75,36.83 53.75,19.05 53.37,18.67 LCD1.1 | v42.57,57.68 41.78,57.68 40.41,59.06 40.41,62.99 39.78,63.63 31.78,63.63 29.04,60.89 MSP1.57
  Bottom 0.203: v42.57,57.68 v48.41,57.68
L8
  Top 0.203: LCD1.20 5.11,16.89 4.22,17.78 4.22,36.58 12.98,45.34 15.52,45.34 16.54,46.36 20.47,46.36 24.66,50.55 24.66,52.83 25.43,53.59 25.43,55.37 29.54,59.48 MSP1.56
L9
  Top 0.203: LCD1.19 7.65,15.11 4.72,18.03 4.72,36.45 13.23,44.96 15.77,44.96 16.79,45.97 20.6,45.97 25.04,50.42 25.04,52.58 25.81,53.34 25.81,55.12 30.04,59.35 MSP1.55
L10
  Top 0.203: LCD1.18 10.19,13.34 5.36,18.16 5.36,36.32 13.61,44.58 16.03,44.58 16.92,45.47 20.65,45.47 21.23,46.05 24.79,49.66 25.55,50.42 25.55,52.32 26.19,52.96 26.19,54.99 30.54,59.34 MSP1.54
L11  (via drill 0.3)
  Top 0.203: LCD1.17 12.73,15.11 9.04,18.67 9.04,37.34 14.38,42.67 21.23,42.67 23.65,45.09 v25.3,45.09 | MSP1.53 31.04,59.21 26.57,54.74 26.57,52.71 26.44,52.58 v26.44,51.94
  Bottom 0.203: v25.3,45.09 25.3,50.8 v26.44,51.94
L12  (via drill 0.3)
  Top 0.203: LCD1.16 15.27,13.72 11.46,17.53 11.46,38.48 14.76,41.78 21.49,41.78 23.65,43.94 25.93,43.94 v26.57,44.58 | MSP1.52 31.54,59.2 27.2,54.86 v27.2,52.96
  Bottom 0.203: v27.2,52.96 27.2,51.56 25.81,50.17 25.81,45.59 26.57,44.83 v26.57,44.58
L13  (via drill 0.3)
  Top 0.203: MSP1.51 32.03,59.18 27.84,54.99 v27.84,52.07 | v27.91,44.12 26.95,43.18 24.03,43.18 21.87,41.02 15.65,41.02 14,39.37 14,16.51 17.81,12.7 LCD1.15
  Bottom 0.203: v27.84,52.07 27.84,51.56 26.31,50.04 26.31,45.72 v27.91,44.12
L14  (via drill 0.3)
  Top 0.203: MSP1.50 32.54,59.06 28.6,55.12 v28.6,52.83 | v28.73,43.18 27.97,42.42 24.28,42.42 22.12,40.26 16.28,40.26 15.65,39.62 15.65,37.08 16.54,36.2 16.54,16.51 20.35,12.7 LCD1.14
  Bottom 0.203: v28.6,52.83 28.6,51.44 26.82,49.66 26.82,46.23 28.73,44.32 v28.73,43.18
L15  (via drill 0.3)
  Top 0.203: 33.05,60.19 33.05,58.93 29.49,55.37 v29.49,51.94 | LCD1.13 22.89,12.7 19.08,16.51 19.08,36.07 21.23,38.23 23.14,38.23 25.32,40.41 29.64,40.41 30.51,41.28 v30.51,41.3 | 33.05,60.2 33.05,60.19 | 33.05,60.19 MSP1.49
  Bottom 0.203: v30.51,41.3 30.35,41.43 29.36,42.42 29.36,44.32 27.33,46.36 27.33,49.53 29.24,51.44 v29.49,51.94
L16  (via drill 0.3)
  Top 0.203: LCD1.12 24.28,11.3 24.16,36.96 26.19,38.99 34.44,38.99 39.01,43.56 v39.01,51.69 | v43.08,51.69 44.35,52.96 44.35,55.5 42.82,57.02 41.81,57.02 40.6,58.23 MSP1.48
  Bottom 0.203: v43.08,51.69 v39.01,51.69
L17  (via drill 0.3)
  Top 0.203: LCD1.11 26.7,11.43 26.7,36.96 28.35,38.61 34.82,38.61 39.65,43.43 39.65,52.07 39.01,52.71 v39.01,53.59 | MSP1.47 40.46,57.73 41.55,56.64 42.57,56.64 43.71,55.5 v43.71,53.72
  Bottom 0.203: v39.01,53.59 43.59,53.59 v43.71,53.72
L18  (via drill 0.3)
  Top 0.203: v43.08,52.96 43.08,55.5 42.44,56.13 41.3,56.13 40.2,57.23 MSP1.46 | LCD1.10 29.24,11.43 29.24,36.96 30.38,38.1 34.82,38.1 40.03,43.31 40.03,52.71 v39.78,52.96
  Bottom 0.203: v43.08,52.96 v39.78,52.96
L19
  Top 0.203: MSP1.45 40.07,56.73 41.43,55.37 41.43,42.16 36.86,37.59 36.86,9.27 36.35,8.76 33.55,8.76 33.05,9.27 LCD1.9
L20
  Top 0.203: MSP1.44 39.55,56.23 41.05,54.74 41.05,42.55 34.32,35.94 34.32,11.43 LCD1.8
L21
  Top 0.203: MSP1.43 39.54,55.73 40.54,54.74 40.54,43.05 34.95,37.47 33.17,37.47 31.78,36.07 31.78,9.65 33.3,8.13 36.6,8.13 38.13,9.65 LCD1.7
L22  (via drill 0.3)
  Top 0.203: LCD1.6 40.67,13.08 39.4,14.35 39.4,37.21 41.81,39.62 41.81,54.86 v42.27,55.35 | MSP1.42 34.99,55.24 38.76,55.24 v39.01,54.99
  Top 0.406: v39.01,54.99
  Bottom 0.203: v39.01,54.99 41.93,54.99 42.27,55.32 | 42.27,55.32 42.32,55.37 | v42.27,55.35 42.27,55.32
L23  (via drill 0.3)
  Top 0.203: LCD1.5 43.21,15.49 41.94,16.76 41.94,38.86 42.44,39.37 v42.44,54.36 | MSP1.41 38.38,54.73 38.76,54.36 v39.78,54.36
  Bottom 0.203: v42.44,54.36 v39.78,54.36
L24
  Top 0.203: LCD1.27 22.89,36.45 25.93,39.5 34.32,39.5 38.38,43.56 38.38,53.59 37.74,54.23 MSP1.40
L25
  Top 0.203: LCD1.26 21.11,35.56 25.55,40.01 34.19,40.01 38,43.82 38,53.21 37.48,53.73 MSP1.39
L26
  Top 0.203: LCD1.25 20.85,38.61 22.89,38.61 25.17,40.89 29.24,40.89 30.89,42.55 36.09,42.55 37.62,44.07 37.62,52.83 37.22,53.23 MSP1.38
L36
  Top 0.203: LCD1.24 15.27,40.13 15.77,40.64 22,40.64 24.16,42.8 27.46,42.8 29.24,44.58 30,44.58 31.04,45.62 MSP1.28
L37
  Top 0.203: LCD1.23 12.73,38.74 15.39,41.4 21.62,41.4 23.77,43.56 26.44,43.56 27.84,44.96 29.74,44.96 30.54,45.75 MSP1.27
L38
  Top 0.203: LCD1.22 10.19,37.85 14.5,42.16 21.36,42.16 23.65,44.45 25.55,44.45 26.44,45.34 29.36,45.34 30.04,46.01 MSP1.26
L39
  Top 0.203: LCD1.21 7.65,36.45 14.25,43.05 20.98,43.05 23.65,45.72 28.98,45.72 29.54,46.28 MSP1.25
N$1
  Top 0.203: 32.66,97.03 32.82,97.18 | 32.82,97.18 32.92,97.28 | R101.1 32.66,97.28 | 32.66,97.28 | 32.82,97.18 LED101.A 32.66,97.27 32.66,97.28
N$2
  Top 0.203: R102.1 32.14,98.41 32.73,99 | 32.73,99 32.79,99.06 | LED102.A 32.73,99
N$4
  Top 0.254: C1.1 18.82,61.09 | MSP1.1 22.18,58.23 19.33,61.09 18.95,61.09
  Top 0.406: C1.1 18.95,61.09
N$6
  Top 0.203: R4.1 27.46,5.59 JP1.2
N$7
  Top 0.203: R4.2 24.37,5.55 23.9,5.08 23.9,4.18 LED1.A
N$8
  Top 0.203: LED2.A 34.73,5.01 R5.2
N$10
  Top 0.254: MSP1.2 22.05,57.73 19.71,60.07 18.91,60.07 C2.1
N$11
  Top 0.254: MSP1.4 21.14,56.73 19.96,57.91 18.94,57.91 C4.1
N$12
  Top 0.305: R119.1 45.53,89.75 45.87,89.41 46.76,89.41 46.78,89.39 T102.2
N$13
  Top 0.254: T102.1 D101.2 D101.1 46.27,94.88 45.87,94.49 44.98,94.49 R118.1
  Top 0.305: R118.1 44.79,94.5
N$14
  Top 0.203: 19.86,55.25 Y1.P2 | Y1.P2 19.47,55.36 18.9,55.93 18.9,56.43 C5.1 | MSP1.6 20.83,55.73 20.35,55.25 19.99,55.25 Y1.P2
N$15
  Top 0.635: L101.1 53.23,86.64 53.23,86.74 | 53.23,86.74 53.24,87.76 53.24,88.27 52.48,89.03 T101.3 | D102.3 48.68,87 49.17,87.5 52.35,87.5 53.11,86.74 53.23,86.74
N$16
  Top 0.203: T102.3 48.8,90.03 48.29,90.55 48.29,93.73 48.79,94.23 49.68,94.23 49.96,93.96 R120.2 | T101.1 50.38,89.73 50.06,90.04 T102.3 | 48.79,90.04 T102.3
  Top 0.406: 48.79,94.23 D101.3
N$17
  Top 0.254: MSP1.5 20.88,56.23 19.96,57.15 18.6,57.15 C4.2
N$18
  Top 0.203: 19.84,54.23 19.91,54.31 19.96,54.31 19.95,54.29 Y1.P1 | Y1.P1 19.52,54.29 18.87,53.65 C6.1 | Y1.P1 20.41,54.29 21.36,55.25 23.57,55.25 MSP1.7
N$19
  Top 0.203: 18.79,58.98 C3.1
  Top 0.254: MSP1.3 21.74,57.23 19.99,58.98 18.91,58.98 C3.1
P1.0/TXD  (via drill 0.3)
  Top 0.203: v11.84,13.34 6.38,18.8 6.38,35.81 14.25,43.69 v16.92,43.69 20.98,43.69 23.67,46.38 v28.7,46.38 29.03,46.71 29.03,47.09 29.04,47.32 MSP1.24 | v13.87,13.34 13.87,9.27 14.63,8.51 28.09,8.51 29.24,7.37 JP1.1 | J1.4 7.77,54.48 7.77,53.21 10.44,50.55 13.49,50.55 v14.12,49.91 | v39.27,62.61 38.89,62.23 37.62,62.23 31.14,55.75 v31.14,52.07 | v41.17,71.12 41.17,71.25 42.06,72.14 42.95,72.14 J101.8
  Bottom 0.203: v11.84,13.34 v13.87,13.34 | v39.27,62.61 41.17,64.52 v41.17,71.12 | v31.14,52.07 31.14,51.69 28.73,49.28 28.73,46.36 v28.7,46.38 | v14.12,49.91 14.12,48.77 16.15,46.74 16.15,44.45 v16.92,43.69
P1.1/RXD  (via drill 0.3)
  Top 0.203: v17.68,44.32 20.85,44.32 23.55,47.02 v28.04,47.02 28.54,47.51 MSP1.23 | J1.3 8.41,56.39 8.41,53.34 10.82,50.93 14.12,50.93 v15.14,49.91 | v38.38,62.99 37.74,62.99 30.33,55.58 v30.33,52.81 | v40.54,70.36 40.54,71.37 41.94,72.77 J101.10
  Bottom 0.203: v38.38,62.99 38.76,62.99 40.54,64.77 v40.54,70.36 | v30.33,52.81 30.33,51.77 27.97,49.4 27.97,47.07 v28.04,47.02 | v17.68,44.32 17.17,44.32 16.66,44.83 16.66,46.99 15.14,48.51 v15.14,49.91
P1.2
  Top 0.203: 28.04,48.2 MSP1.22 28.09,48.73 28.09,48.39 28.04,48.34 28.04,47.98 27.69,47.62 23.52,47.62 20.85,44.96 17.17,44.96 16.41,44.2 14,44.2 5.87,36.07 5.87,18.29 11.46,12.7 11.46,7.02 11.47,7.02 S1.4 11.46,6.87 11.46,6.98 20.07,6.98 S1.3
P1.3  (via drill 0.3)
  Top 0.203: MSP1.21 27.54,49.61 27.71,49.78 33.43,49.78 33.81,49.4 33.81,47.75 34.57,46.99 v35.2,46.99
  Bottom 0.203: 52.22,45.72 J2.8 50.83,46.99 48.79,46.99 48.54,46.74 47.14,46.74 46.89,46.99 v35.2,46.99
P1.4  (via drill 0.3)
  Top 0.203: v48.16,47.37 48.16,43.94 48.79,43.31 51.97,43.31 J2.9 | MSP1.20 27.04,49.62 27.58,50.17 33.55,50.17 34.19,49.53 34.19,48.13 34.7,47.62 v35.97,47.62
  Bottom 0.203: v35.97,47.62 47.02,47.62 47.27,47.37 v48.16,47.37
P1.5  (via drill 0.3)
  Top 0.203: J2.10 50.57,40.64 47.52,43.69 v47.52,48.26 | MSP1.19 26.54,49.75 27.33,50.55 33.81,50.55 34.57,49.78 34.57,48.51 34.82,48.26 v35.2,48.26
  Bottom 0.203: v35.2,48.26 v47.52,48.26
P1.6  (via drill 0.3)
  Top 0.203: J2.3 49.56,60.96 v47.78,60.96 | v39.65,60.2 37.49,60.2 v36.73,59.44 | MSP1.18 26.04,49.89 27.08,50.93 32.41,50.93 33.05,51.56 33.05,55.63 v33.3,55.88
  Bottom 0.203: v39.65,60.2 40.41,60.96 v47.78,60.96 | v33.3,55.88 v36.73,59.44
P1.7  (via drill 0.3)
  Top 0.203: J2.2 51.46,61.6 v46.51,61.6 | MSP1.17 25.54,49.9 26.95,51.31 32.16,51.31 32.41,51.56 32.41,56.01 v33.3,56.9 | v39.52,61.21 37.62,61.21 v35.71,59.31
  Bottom 0.203: v33.3,56.9 v35.71,59.31 | v46.51,61.6 40.41,61.6 39.9,61.6 v39.52,61.21
P2.3/RTS  (via drill 0.3)
  Top 0.203: v43.46,66.17 45.49,64.14 45.49,61.72 49.05,58.17 v49.05,52.88 | v43.46,68.71 37.49,68.71 36.86,69.34 J101.14 | 35.08,52.71 35.05,52.73 MSP1.37 35.01,52.71 36.09,52.71 36.2,52.6 v36.55,52.6
  Bottom 0.203: v43.46,66.17 v43.46,68.71 | v49.05,52.88 49.05,52.83 48.54,52.32 38,52.32 37.69,52.63 v36.55,52.6
P2.4/CTS  (via drill 0.3)
  Top 0.203: v47.65,51.46 47.65,58.93 45.11,61.47 45.11,63.63 42.7,66.04 v42.7,66.68 | v42.7,69.34 39.9,69.34 39.4,69.85 J101.12 | MSP1.36 35.04,52.23 35.08,52.2 35.97,52.2 36.4,51.77 v36.98,51.77
  Bottom 0.203: v42.7,66.68 v42.7,69.34 | v47.65,51.46 47.24,51.05 37.69,51.05 v36.98,51.77
P2.5  (via drill 0.3)
  Top 0.203: J1.8 6.63,45.97 v14.12,45.97 | MSP1.35 35.8,51.73 36.35,51.18 36.73,51.18 37.11,50.8 37.11,44.2 35.84,42.93 30.63,42.93 28.98,41.28 24.92,41.28 22.63,38.99 18.44,38.99 17.68,38.23 v16.54,38.23
  Bottom 0.203: v16.54,38.23 14.63,40.13 14.63,45.47 v14.12,45.97
P2.6  (via drill 0.3)
  Top 0.203: S2.4 46.09,6.87 46.15,6.93 46.17,6.93 S2.3 46.76,6.86 46.76,6.6 44.48,8.89 44.48,37.85 43.33,38.99 43.33,50.04 v43.71,50.42 | MSP1.34 35.66,51.23 36.47,50.42 v36.5,50.42
  Bottom 0.203: v43.71,50.42 v36.5,50.42
P2.7  (via drill 0.3)
  Top 0.203: J1.5 6.88,53.34 10.31,49.91 v13.11,49.91 | MSP1.33 35.53,50.73 35.84,50.42 35.84,50.04 36.6,49.28 36.6,44.32 35.59,43.31 30.38,43.31 28.73,41.66 24.66,41.66 22.5,39.5 17.81,39.5 v17.55,39.24
  Bottom 0.203: v17.55,39.24 15.77,41.02 15.77,46.36 13.11,49.02 v13.11,49.91
P4.0
  Top 0.203: R5.1 32.93,5.72 31.9,5.72 31.27,5.08 31.27,3.3 30.38,2.41 23.77,2.41 20.73,5.46 9.68,5.46 8.15,6.98 4.85,6.98 3.58,8.26 3.58,50.42 5.11,51.94 7.52,51.94 10.19,49.28 20.09,49.28 20.98,50.17 20.98,51.31 22.41,52.73 MSP1.12
P5.0  (via drill 0.3)
  Top 0.203: v49.05,46.36 49.05,48.51 50.06,49.53 50.06,54.61 51.33,55.88 J2.4 | MSP1.32 33.04,47.38 34.06,46.36 35.08,46.36 35.08,46.35 v35.96,46.35 v35.97,46.36
  Bottom 0.203: v35.97,46.36 v49.05,46.36
P5.1  (via drill 0.3)
  Top 0.203: v16.54,39.24 17.04,39.88 22.25,39.88 24.54,42.04 28.47,42.04 30.38,43.94 v33.93,43.94 | J1.7 8.03,46.61 14.5,46.61 v15.14,45.97 | MSP1.31 32.54,46.61 33.43,45.72 v33.93,45.72
  Bottom 0.203: v33.93,45.72 v33.93,43.94 | v15.14,45.97 15.14,40.64 v16.54,39.24
P5.2  (via drill 0.3)
  Top 0.203: v49.81,45.72 49.81,48.51 J2.6 | v34.95,45.72 34.19,44.96 33.43,44.96 32.04,46.35 MSP1.30
  Bottom 0.203: v34.95,45.72 v49.81,45.72
P5.3  (via drill 0.3)
  Top 0.203: J2.7 50.44,46.61 50.44,45.47 50.06,45.09 v48.79,45.09 | v35.84,45.09 35.2,45.09 34.7,44.58 33.17,44.58 31.54,46.21 MSP1.29
  Bottom 0.203: v35.84,45.09 v48.79,45.09
P8.0
  Top 0.203: J1.6 10.19,46.99 20.35,46.99 22.76,49.4 22.76,50.42 23.07,50.73 MSP1.16
P8.1  (via drill 0.3)
  Top 0.203: v11.07,51.56 8.92,53.72 8.92,58.42 J1.2 | v13.23,47.62 20.35,47.62 22.25,49.53 22.25,50.67 22.81,51.23 MSP1.15
  Bottom 0.203: v13.23,47.62 13.23,48.26 12.34,49.15 12.34,51.05 11.84,51.56 v11.07,51.56
P8.2  (via drill 0.3)
  Top 0.203: v11.96,45.21 9.93,45.21 7.9,43.18 J1.9 | v11.96,47.62 12.6,48.26 20.35,48.26 21.87,49.78 21.87,50.93 22.68,51.73 MSP1.14
  Bottom 0.203: v11.96,47.62 v11.96,45.21
P8.3  (via drill 0.3)
  Top 0.203: v10.95,47.62 12.09,48.77 20.22,48.77 21.49,50.04 21.49,51.18 22.54,52.23 MSP1.13 | v10.95,44.58 10.31,44.58 J1.10
  Bottom 0.203: v10.95,47.62 v10.95,44.58
RST/SBWTDIO  (via drill 0.3)
  Top 0.203: 47.02,74.04 J101.6 47.02,68.83 v46.25,68.07 22.76,68.07 19.14,64.45 v18.89,64.45 C11.1 R1.2 18.94,62.1 21.11,62.1 24.66,58.55 24.66,54.1 24.29,53.73 MSP1.10 | J2.5 54.64,55.88 54.64,64.26 52.22,66.68 v46.25,66.68 | S3.3 S3.4 16.14,67.68 v16.54,68.07
  Bottom 0.203: v46.25,66.68 v46.25,68.07 | v18.89,64.45 16.54,66.8 v16.54,68.07
TEST/SBWTCK
  Top 0.203: J101.4 49.43,73.53 49.43,68.33 48.54,67.44 27.84,67.44 25.04,64.64 25.04,53.85 24.43,53.23 MSP1.11

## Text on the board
tPlace: RST | 1 | 21 | 20 | 10 | 11 | P5.7 | P5.6 | P5.5 | P5.4 | P2.2 | P2.1 | P2.0 | NC | NC | NC | NC | NC | NC | NC | P7.0 | P7.1 | P7.2 | P7.3 | P3.0 | P3.1 | P3.2 | P3.3 | P3.4 | P3.5 | P3.6 | P3.7 | P6.0 | P6.1 | P6.2 | P6.3 | P6.4 | P6.5 | P6.6 | P6.7 | P7.4 | P7.5 | P7.7 | P7.6 | GND | GND | 3V3 | P1.0 | P4.0 | P1.2 | P2.6
tDocu: IC103 | eZ-FET Rev1.2 | Rev 1.0 | MSP-EXP430FR4133 | GND | 5V | 3V3 | RTS >> | CTS << | RXD << | TXD >> | SBWTDIO | SBWTCK | 5V | GND | P8.1 | PWM | A9 | P1.7 | P1.1 | I/O! | RXD | P1.6 | P1.0 | I/O | TXD | P5.0 | P2.7 | I/O! | !RST | P8.0 | MOSI | A8 | P5.2 | P5.1 | MISO | SCLK | P5.3 | P2.5 | I/O! | I/O! | P1.3 | P8.2 | I/O! | SCL | * | P1.4 | P8.3 | * | I/O! | SDA | P1.5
